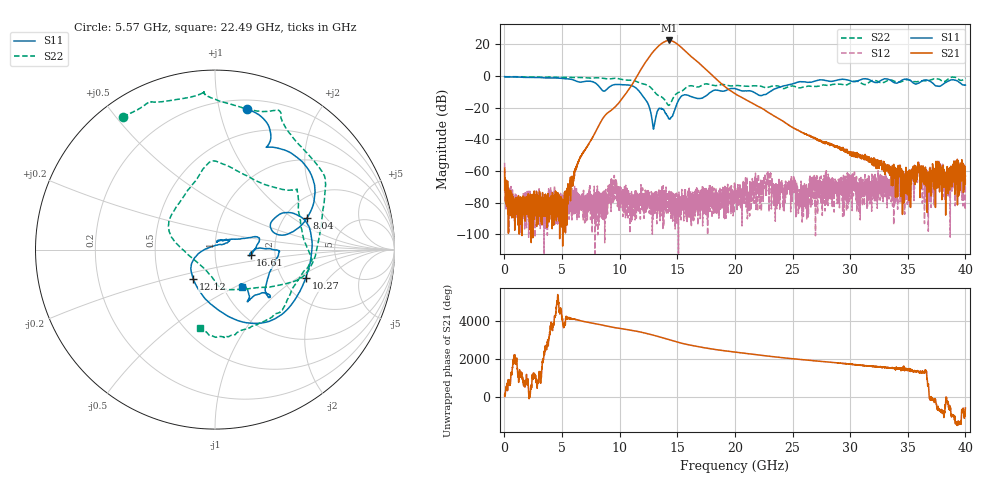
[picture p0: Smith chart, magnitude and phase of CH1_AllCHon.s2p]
!Keysight Technologies,N5245B,MY57181321,A.14.80.03
!Date: Thursday, August 24, 2023 18:40:36
!Correction: S11(C  2-Port  )
!S21(C  2-Port  )
!S12(C  2-Port  )
!S22(C  2-Port  )
!S2P File: Measurements: S11, S21, S12, S22:
# Hz S  RI  R 50
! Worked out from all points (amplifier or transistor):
!   4000 points, 10 MHz to 40 GHz, reference 50 ohm
!   highest |S21| = 22.5 dB at 14.3 GHz (marker M1)
!   |S21| within 3 dB of that: 13.45 GHz to 15.12 GHz (1.672 GHz wide, 11.7 % of centre)
!   unconditionally stable (mu >= 1): start of sweep to end of sweep
!   at 6.67 GHz: K = 244504.23, MAG = -40.8 dB, |S12| = -82.3 dB
!   at 20.01 GHz: K = 4769.91, MAG = -9.2 dB, |S12| = -72.4 dB
!   at 40 GHz: K = 203894.01, MAG = -55.8 dB, |S12| = -63.8 dB
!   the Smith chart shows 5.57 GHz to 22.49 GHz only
!   S11 on the Smith chart (normalised r, x): 5.57 GHz: 0.28, +1.22; 8.04 GHz: 2.63, +1.32; 10.27 GHz: 2.67, -1.18; 12.12 GHz: 0.75, -0.26; 16.61 GHz: 1.49, -0.10; 22.49 GHz: 1.22, -0.55
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1e7  -0.9465 0.0482  -0.000342 0.00118  0.000638 -0.0017  -0.9505 0.0226
5.57e9  0.1798 0.7833  -0.000328 5.22e-05  0.000106 0.000181  -0.5121 0.7395
6.68e9  0.2976 0.5709  0.00269 0.00135  -8.03e-05 -0.000127  -0.3522 0.8228
8.04e9  0.5128 0.1768  -0.0142 -0.0161  -0.000133 6.89e-05  -0.0626 0.8776
1.027e10  0.5057 -0.1585  0.181 -0.0964  -3.24e-05 1.63e-05  0.4213 0.6421
1.212e10  -0.1203 -0.1657  -1.277 1.957  -5.45e-05 5.57e-05  0.5514 -0.0554
1.272e10  -0.0634 -0.00212  3.973 2.698  -5.29e-05 -2.76e-06  0.3745 -0.1943
1.334e10  0.0734 0.0434  3.272 -8.01  -7.48e-05 0.000102  0.0966 -0.2233
1.363e10  0.0792 0.0492  -4.978 -9.329  -4.82e-05 0.000222  0.0315 -0.2158
1.392e10  0.049 0.0527  -12.1 -2.166  0.000116 -0.000136  -0.00239 -0.173
1.43e10  0.0114 0.0436  -6.622 11.51  0.000112 0.000201  -0.0934 -0.0761
1.456e10  0.0219 0.0484  3.864 12.09  0.000158 -3e-05  -0.1766 -0.00246
1.491e10  0.1024 0.0584  10.54 2.278  -4.19e-05 -6.03e-05  -0.2552 0.0992
1.547e10  0.2337 0.0713  2.043 -6.987  2.92e-05 4.99e-05  -0.1688 0.3047
1.597e10  0.2404 0.0349  -3.704 -3.173  3.06e-05 -2.39e-05  -0.0433 0.4746
1.661e10  0.1983 -0.0307  -2.556 1.778  2.88e-05 3.92e-05  0.1309 0.4343
1.762e10  0.2558 0.00845  1.178 0.8492  0.000138 -0.000167  0.4593 0.322
2.001e10  0.3077 -0.2576  -0.2603 -0.0847  -0.000169 -0.000172  0.3865 -0.3162
2.249e10  0.1505 -0.2093  0.0858 0.0226  0.000338 -0.000259  -0.0825 -0.4394
2.667e10  0.1323 -0.6302  -0.00532 0.011  -4.16e-05 7.48e-05  -0.3231 0.3482
3.334e10  -0.6941 -0.3609  0.000197 0.00105  7.73e-05 0.000479  0.7297 -0.099
4e10  -0.0687 0.5112  -0.000624 0.000304  0.000159 0.000622  0.3496 -0.7938
